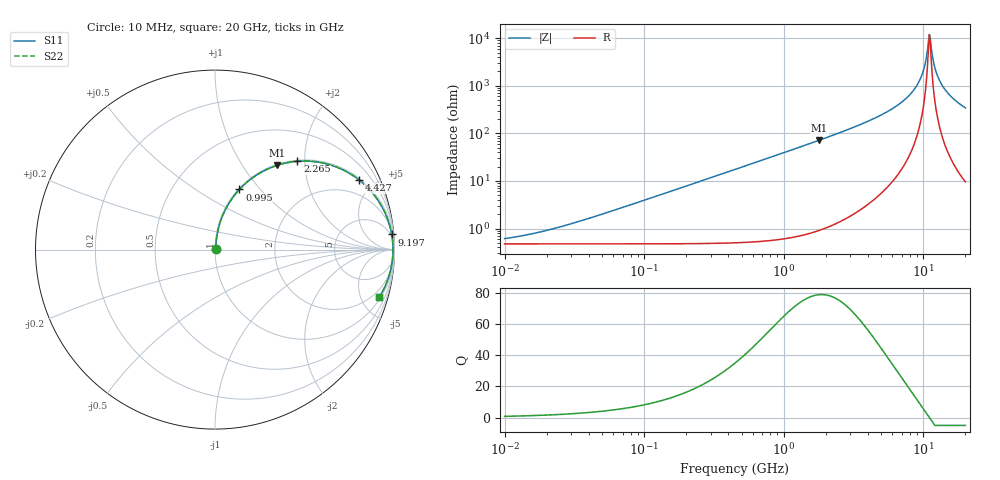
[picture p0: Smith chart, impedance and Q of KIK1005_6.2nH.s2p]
!version-3
!date-01.2023
!Series
# Hz S RI R 50
!Freq ReS11 ImS11 ReS21 ImS21 ReS12 ImS12 ReS22 ImS22
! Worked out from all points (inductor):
!   500 points, 10 MHz to 20 GHz, reference 50 ohm
!   read as one part in series: L = 6.2 nH near 37.06 MHz
!   highest Q = 78.7 at 1.802 GHz (marker M1), where L = 6.37 nH
!   self-resonance near 11.04 GHz
!   S11 on the Smith chart (normalised r, x): 10 MHz: 1.01, +0.01; 995 MHz: 1.01, +0.78; 2.265 GHz: 1.02, +1.84; 4.427 GHz: 1.08, +4.10; 9.197 GHz: 3, +23; 20 GHz: 1.19, -6.88
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1e7  0.00473 0.00386  0.9953 -0.00386  0.9953 -0.00386  0.00473 0.00386
1.783943e7  0.00477 0.00688  0.9952 -0.00688  0.9952 -0.00688  0.00477 0.00688
3.59488e7  0.00491 0.0139  0.9951 -0.0139  0.9951 -0.0139  0.00491 0.0139
1.272781e8  0.00716 0.049  0.9928 -0.049  0.9928 -0.049  0.00716 0.049
4.506326e8  0.0345 0.1689  0.9655 -0.1689  0.9655 -0.1689  0.0345 0.1689
9.949878e8  0.1363 0.3355  0.8637 -0.3355  0.8637 -0.3355  0.1363 0.3355
1.595481e9  0.2896 0.4472  0.7104 -0.4472  0.7104 -0.4472  0.2896 0.4472
1.802246e9  0.344 0.4687  0.656 -0.4687  0.656 -0.4687  0.344 0.4687
2.264871e9  0.4594 0.4919  0.5406 -0.4919  0.5406 -0.4919  0.4594 0.4919
4.427068e9  0.8035 0.3877  0.1965 -0.3877  0.1965 -0.3877  0.8035 0.3877
5.648861e9  0.8921 0.2972  0.1079 -0.2972  0.1079 -0.2972  0.8921 0.2972
7.544864e9  0.9602 0.1734  0.0398 -0.1734  0.0398 -0.1734  0.9602 0.1734
9.197084e9  0.9845 0.0844  0.0155 -0.0844  0.0155 -0.0844  0.9845 0.0844
1.007725e10  0.9899 0.0428  0.0101 -0.0428  0.0101 -0.0428  0.9899 0.0428
1.087473e10  0.9917 0.0081  0.00826 -0.0081  0.00826 -0.0081  0.9917 0.0081
1.104164e10  0.9918 0.00115  0.00818 -0.00115  0.00818 -0.00115  0.9918 0.00115
1.13832e10  0.9917 -0.0128  0.00833 0.0128  0.00833 0.0128  0.9917 -0.0128
1.191544e10  0.9907 -0.0336  0.00929 0.0336  0.00929 0.0336  0.9907 -0.0336
1.228403e10  0.9896 -0.0475  0.0104 0.0475  0.0104 0.0475  0.9896 -0.0475
1.345961e10  0.9838 -0.0891  0.0162 0.0891  0.0162 0.0891  0.9838 -0.0891
1.591478e10  0.9639 -0.1646  0.0361 0.1646  0.0361 0.1646  0.9639 -0.1646
2e10  0.9159 -0.2641  0.0841 0.2641  0.0841 0.2641  0.9159 -0.2641
